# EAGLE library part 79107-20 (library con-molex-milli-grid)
RECEPTACAL
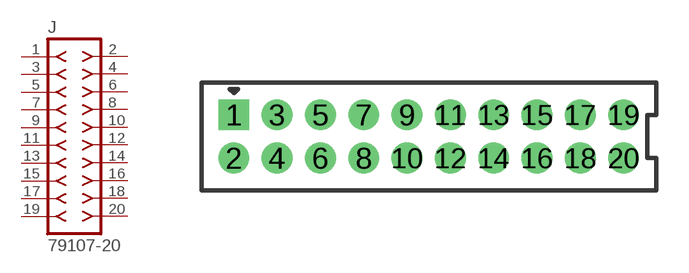
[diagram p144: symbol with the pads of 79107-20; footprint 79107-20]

Designator prefix J

## 79107-20  [79107-20]
1  1  pas
2  2  pas
3  3  pas
4  4  pas
5  5  pas
6  6  pas
7  7  pas
8  8  pas
9  9  pas
10  10  pas
11  11  pas
12  12  pas
13  13  pas
14  14  pas
15  15  pas
16  16  pas
17  17  pas
18  18  pas
19  19  pas
20  20  pas

## Footprint 79107-20 (pad centres in mm)
RECEPTACAL Dual Row, Vertical, Through-Hole
drill 0.914 square: 1 -9,1
drill 0.914: 2 -9,-1; 3 -7,1; 4 -7,-1; 5 -5,1; 6 -5,-1; 7 -3,1; 8 -3,-1; 9 -1,1; 10 -1,-1; 11 1,1; 12 1,-1; 13 3,1; 14 3,-1; 15 5,1; 16 5,-1; 17 7,1; 18 7,-1; 19 9,1; 20 9,-1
